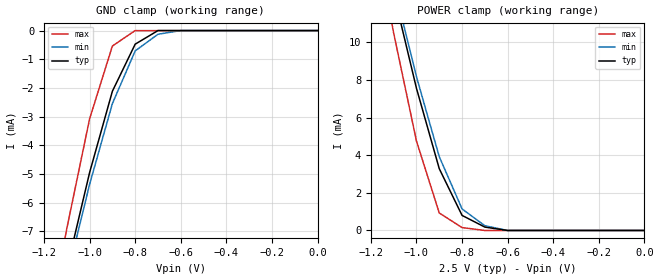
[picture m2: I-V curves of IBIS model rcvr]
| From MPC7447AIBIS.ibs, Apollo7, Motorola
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| *   rcvr  Model   *
[Model]   rcvr
Model_type   Input
Polarity   Non-Inverting
Vinl =   0.87V
Vinh =   1.63V
|   typ   min   max
C_comp   1.454738e-12   1.068448e-12   1.585284e-12
|   typ   min   max
[Voltage range]   2.5V   2.3V   2.7V
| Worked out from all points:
|   GND clamp passes 1 mA (typ) near -0.83 V on its own axis
|   POWER clamp passes 1 mA (typ) near -0.81 V on its own axis
|   Voltage(V)   I(typ)   I(min)   I(max)
[GND_clamp]
-2.5V     -62.89mA   -61.15mA   -71.54mA
-1.2V     -11.91mA   -12.08mA   -11.14mA
-1.1V     -8.313mA   -8.62mA    -6.904mA
-1V       -4.952mA   -5.364mA   -3.078mA
-900mV    -2.115mA   -2.545mA   -537.7uA
-800mV    -473.7uA   -709.1uA   0A
-700mV    0A         -127.9uA   0A
-600mV    0A         0A         0A
0V        0A         0A         0A
[POWER_clamp]
-2.5V     94.61mA    92.19mA    107.2mA
-1.2V     18mA       18.29mA    16.83mA
-1.1V     12.6mA     13.07mA    10.48mA
-1V       7.549mA    8.167mA    4.747mA
-900mV    3.281mA    3.919mA    928.8uA
-800mV    800.4uA    1.145mA    153.8uA
-700mV    180uA      252.6uA    0A
-600mV    0A         0A         0A
0V        0A         0A         0A
